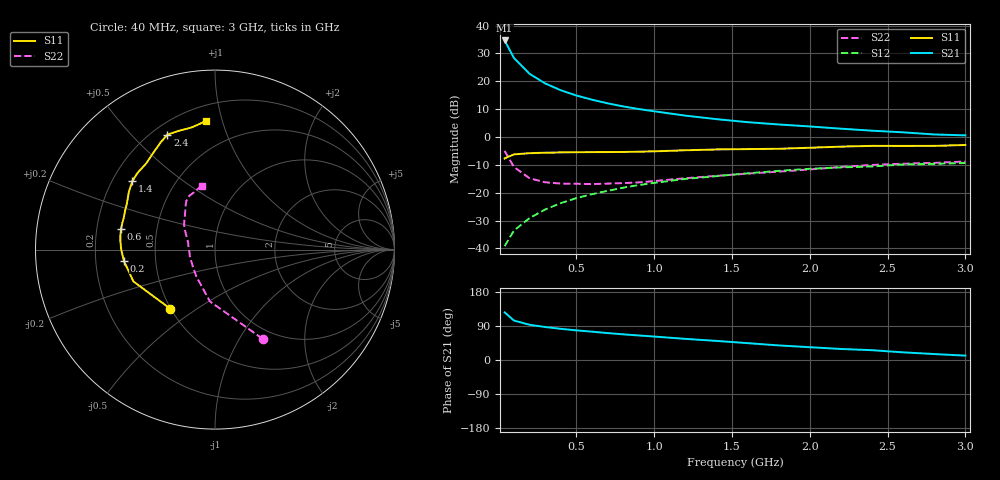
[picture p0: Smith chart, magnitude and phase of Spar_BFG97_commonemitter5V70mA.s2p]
! Filename:  BFG97D.S2P  Version:  2.0
! NXP part #: BFG97  Date: Jul 1990
! Bias condition: Vce=5V, Ic=70mA
#  MHz  S  MA  R  50
! Freq  S11  S21  S12  S22  !GUM [dB]
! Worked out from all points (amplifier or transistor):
!   21 points, 40 MHz to 3 GHz, reference 50 ohm
!   highest |S21| = 34.6 dB at 40 MHz (marker M1)
!   |S21| within 3 dB of that: start of sweep to 68.65 MHz
!   unconditionally stable (mu >= 1): 193.6 MHz to 2.918 GHz
!   at 300 MHz: K = 1.05, MAG = 21.3 dB, |S12| = -26.0 dB
!   at 1 GHz: K = 1.08, MAG = 11.1 dB, |S12| = -16.5 dB
!   at 3 GHz: K = 0.98, MSG = 5.0 dB, |S12| = -9.3 dB
!   S11 on the Smith chart (normalised r, x): 40 MHz: 0.50, -0.40; 200 MHz: 0.32, -0.05; 600 MHz: 0.31, +0.10; 1.4 GHz: 0.28, +0.33; 2.4 GHz: 0.26, +0.64; 3 GHz: 0.30, +0.89
40  0.413 -127.0  54 125.8  0.011 67.6  0.564 -61.9
100  0.488 -158.7  26.2 104.1  0.021 67.1  0.29 -95.6
200  0.512 -173.1  13.63 93.0  0.035 72.1  0.182 -124.9
300  0.523 179.7  9.172 87.1  0.05 72.7  0.154 -144.1
400  0.529 175.0  6.916 82.3  0.065 72.4  0.146 -156.8
500  0.533 171.4  5.563 78.3  0.08 71.9  0.145 -166.6
600  0.536 167.8  4.682 74.8  0.094 70.9  0.143 -174.4
700  0.537 164.0  4.034 71.1  0.108 70.1  0.146 179.4
800  0.539 160.2  3.549 67.8  0.123 68.7  0.149 172.9
900  0.546 156.6  3.181 64.8  0.137 67.3  0.153 166.7
1000  0.553 152.7  2.895 61.9  0.15 66.0  0.162 161.1
1200  0.578 146.1  2.422 55.8  0.177 63.0  0.182 152.5
1400  0.598 140.4  2.092 50.4  0.198 59.7  0.201 146.6
1600  0.607 135.3  1.848 44.5  0.223 57.8  0.22 141.5
1800  0.615 128.4  1.679 38.5  0.247 53.1  0.239 135.5
2000  0.642 122.0  1.547 33.8  0.269 50.7  0.262 129.5
2200  0.672 116.5  1.411 29.1  0.285 47.5  0.29 124.6
2400  0.693 112.5  1.299 25.9  0.296 46.2  0.315 120.5
2600  0.692 107.5  1.213 20.2  0.322 42.1  0.332 115.4
2800  0.693 100.7  1.111 15.7  0.33 37.2  0.343 108.8
3000  0.719 93.8  1.07 11.5  0.342 35.4  0.364 101.8
